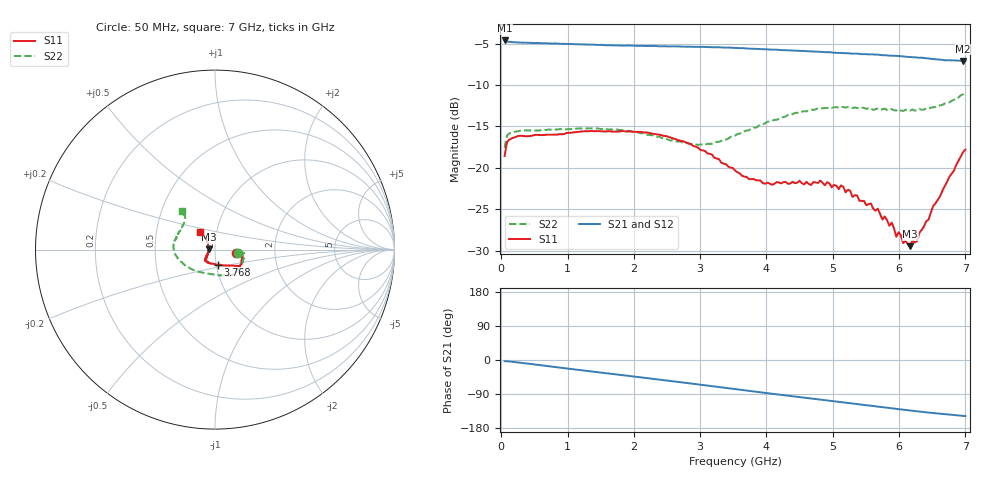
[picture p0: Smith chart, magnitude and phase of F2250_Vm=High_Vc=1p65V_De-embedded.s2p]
! Integrated Device Technology
! Corporate Headquarters
! 6024 Silver Creek Valley Road
! San Jose, CA 95138  USA
! Phone:  1-408-284-8200
! Toll Free:  1-800-223-1366
! Webpage:  http://www.idt.com/
! Timing and RF Division
! 515 Groton Road, Suite 102
! Westford, MA 01886-6024
! Device:  F2250
! Description: Voltage Variable RF Attenuator
! Frequency:  50.0 -  6000.00 MHz
! Package:  3x3 mm Thin QFN Plastic Package: 16 pin
! Ports:  2 RF, 3 DC
!  Pin  1  = GND
!  Pin  2  = NC
!  Pin  3  = RF1  = Port 1
!  Pin  4  = NC
!  Pin  5  = GND
!  Pin  6  = GND
!  Pin  7  = GND
!  Pin  8  = GND
!  Pin  9  = NC
!  Pin 10  = RF2  = Port 2
!  Pin 11  = NC
!  Pin 12  = GND
!  Pin 13  = GND
!  Pin 14  = VCNTRL
!  Pin 15  = VDD
!  Pin 16  = VMODE
! Vcntrl:  1.650 Volts
! Vmode:  +3.300 Volts
! Vdd:  +3.30  Volts
! Current:  1.328 mA
! Data:  The device was measured on a the F2250 evaluation board which has
!  individual transmission lines to the RF pins.  Data was collected
!  using a calibrated network analyzer.  The evaluation board was
!  de-embedded using a TRL calibration technique.
!  The reference plane is the edge of the package pin.
! Misc:  SN 10
!  Action Tracker AT0258
! Date Measured:  2014-11-26
! Date:  2015-10-15  MJV
! Note:
!  Integrated Device Technology supplies this data as a sample of measured
!  data at the package pin for this product.  Your particular data for this
!  product may vary.
!  Data was taken at 25 degrees C.
!  Integrated Device Technology reserves the right to change this data at anytime.
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# GHz S dB R 50
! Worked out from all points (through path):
!   201 points, 50 MHz to 7 GHz, reference 50 ohm
!   highest |S21| = -4.63 dB at 50 MHz (marker M1); lowest = -7.1 dB at 6.965 GHz (marker M2)
!   group delay of S21, straight-line fit = 59.4 ps
!   lowest |S11| = -29.4 dB at 6.166 GHz (marker M3), VSWR 1.07, Z = 46.7 + j0.112 ohm
!   |S11| at or under -10 dB: start of sweep to end of sweep
!   |S22| runs from -17.6 to -11.0 dB; largest |S21 - S12| = 0.0025
!   S11 on the Smith chart (normalised r, x): 50 MHz: 1.26, -0.05; 3.768 GHz: 1.01, -0.17; 7 GHz: 0.83, +0.17
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0.05  -18.55 -9.4  -4.63 -3.2  -4.64 -3.2  -17.59 -9.2
0.08475  -16.92 -5.7  -4.77 -3.3  -4.77 -3.3  -16.11 -6.4
0.2585  -16.14 -7.9  -4.87 -6.6  -4.86 -6.6  -15.57 -11.4
1.2315  -15.58 -27.8  -5.11 -27.5  -5.11 -27.6  -15.21 -43.5
2.37825  -15.99 -35.2  -5.33 -51.6  -5.34 -51.6  -16.22 -70.9
2.969  -17.56 -42.0  -5.41 -64.4  -5.40 -64.4  -17.23 -97.0
3.525  -20.30 -63.9  -5.52 -76.7  -5.52 -76.8  -16.10 -129.7
3.76825  -21.36 -80.2  -5.62 -82.1  -5.61 -82.2  -15.28 -142.0
4.081  -22.03 -99.4  -5.73 -89.0  -5.73 -89.0  -14.34 -155.3
4.7065  -21.70 -127.9  -5.96 -102.5  -5.97 -102.5  -13.00 -174.0
5.1235  -22.11 -136.4  -6.13 -111.4  -6.12 -111.5  -12.67 175.6
5.29725  -23.50 -134.9  -6.22 -115.0  -6.21 -115.1  -12.77 171.9
5.6795  -24.92 -144.0  -6.34 -123.1  -6.36 -123.2  -12.85 162.3
5.85325  -26.98 -150.4  -6.46 -126.7  -6.46 -126.8  -13.02 156.8
5.888  -26.60 -152.3  -6.46 -127.5  -6.46 -127.5  -12.90 156.9
5.9575  -28.30 -157.6  -6.48 -128.9  -6.49 -129.0  -13.07 154.1
5.99225  -27.76 -163.6  -6.50 -129.7  -6.51 -129.8  -12.93 153.6
6.06175  -29.07 -167.4  -6.55 -131.0  -6.55 -131.1  -13.13 150.9
6.166  -29.44 178.0  -6.62 -133.2  -6.64 -133.2  -13.08 147.6
6.27025  -28.84 161.6  -6.68 -135.3  -6.70 -135.4  -13.06 144.2
6.96525  -18.09 130.6  -7.12 -147.5  -7.13 -147.6  -11.13 131.1
7  -17.78 130.5  -7.11 -148.0  -7.12 -148.1  -10.97 130.3
